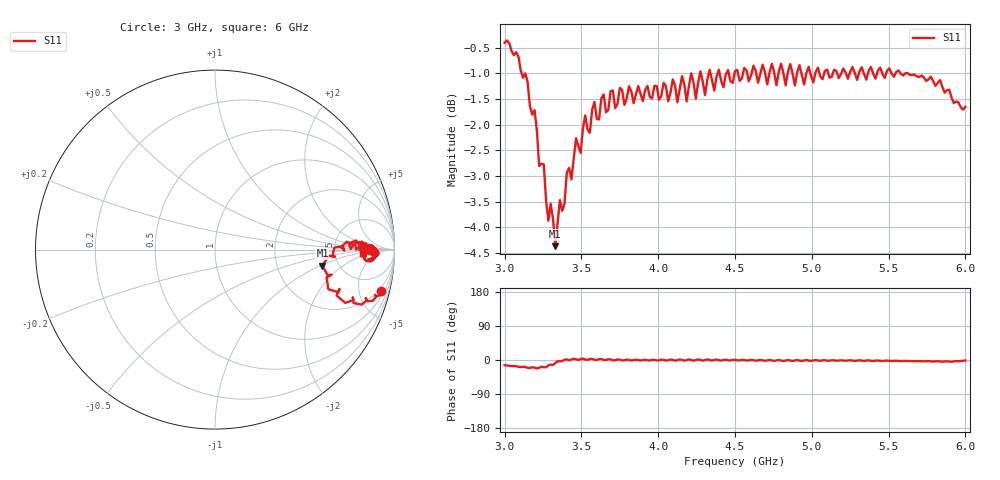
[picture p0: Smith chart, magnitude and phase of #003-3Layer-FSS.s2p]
!  05/08/2025  16:07:21
! Ref Plane: 0.000 mm
# MHZ S MA R  50
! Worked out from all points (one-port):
!   201 points, 3 GHz to 6 GHz, reference 50 ohm
!   lowest |S11| = -4.4 dB at 3.33 GHz (marker M1), VSWR 4.06, Z = 187 - j52.5 ohm
!   |S11| at or under -10 dB: nowhere
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3000  0.9542 -13.9
3135  0.891 -18.5
3210  0.7839 -22.2
3330  0.6048 -8.4
3375  0.6547 -3.1
3450  0.7354 3.5
3525  0.8109 1.4
3555  0.7798 2.8
3585  0.8357 0.7
3750  0.8624 0.9
4065  0.837 -0.7
4095  0.879 0.2
4125  0.835 -0.5
4155  0.8856 0.1
4185  0.8366 -0.3
4215  0.8911 0.1
4245  0.8419 -0.1
4275  0.8951 -0.0
4305  0.8485 0.1
4335  0.8981 -0.1
4365  0.8574 0.1
4500  0.8956 0.3
4875  0.89 -2.7
4905  0.8937 -0.1
5250  0.8941 -0.7
5625  0.8913 -2.8
5910  0.8439 -4.3
6000  0.8266 -1.3
